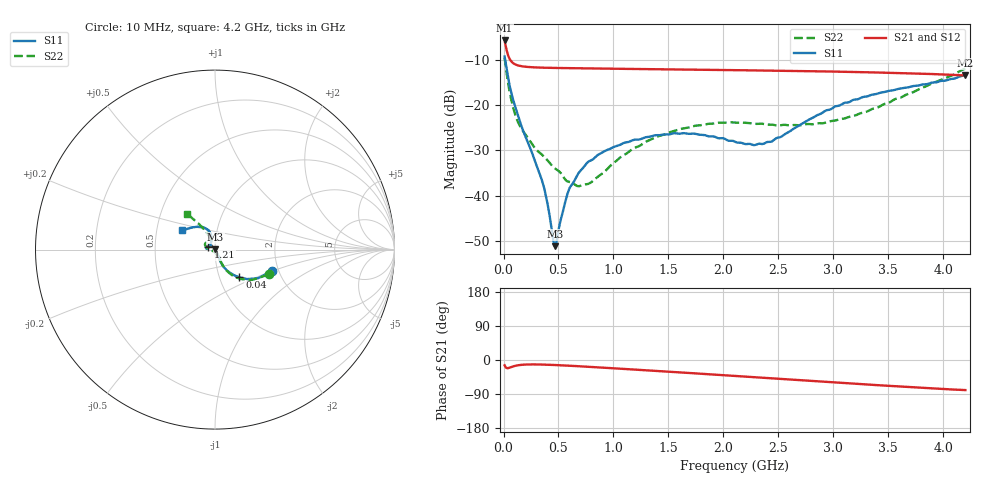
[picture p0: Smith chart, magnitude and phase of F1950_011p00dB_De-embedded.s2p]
! Integrated Device Technology
! Corporate Headquarters
! 6024 Silver Creek Valley Road
! San Jose, CA 95138  USA
! Phone:  1-408-284-8200
! Toll Free:  1-800-223-1366
! Webpage:  http://www.idt.com/
! Timing and RF Division
! 515 Groton Road, Suite 102
! Westford, MA 01886-6024
! Device:  F1950
! Description: 7-bit 0.25 dB Digital Step Attenuator
! Frequency:  150.0 -  4000.00 MHz
! Package:  4x4 mm Thin QFN Plastic Package: 24 pin
! Ports:  2 RF, 12 DC
!  Pin  1  = D0
!  Pin  2  = VDD
!  Pin  3  = Vmode
!  Pin  4  = GND
!  Pin  5  = RF1  =  Port 1
!  Pin  6  = GND
!  Pin  7  = GND
!  Pin  8  = GND
!  Pin  9  = GND
!  Pin 10  = GND
!  Pin 11  = GND
!  Pin 12  = GND
!  Pin 13  = GND
!  Pin 14  = RF2  =  Port 2
!  Pin 15  = GND
!  Pin 16  = LE
!  Pin 17  = CLK
!  Pin 18  = DATE
!  Pin 19  = D6
!  Pin 20  = D5
!  Pin 21  = D4
!  Pin 22  = D3
!  Pin 23  = D2
!  Pin 24  = D1
! State:  44
! Atten State:  11.00 dB
! Voltage:  +5.00 Volts
! Current:  Not Measured mA
! Data:  The device was measured on a the F195X evaluation board which has
!  individual transmission lines to the RF pins.  Data was collected
!  using a calibrated network analyzer.  The evaluation board was
!  de-embedded using a TRL calibration technique.
!  The reference plane is the edge of the package pin.
! Misc:  Board 2019
!  Action Tracker AT0250
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# GHz S dB R 50
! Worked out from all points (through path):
!   420 points, 10 MHz to 4.2 GHz, reference 50 ohm
!   highest |S21| = -5.80 dB at 10 MHz (marker M1); lowest = -13.5 dB at 4.2 GHz (marker M2)
!   group delay of S21, straight-line fit = 48.5 ps
!   lowest |S11| = -51.0 dB at 470 MHz (marker M3), VSWR 1.01, Z = 50.2 + j0.171 ohm
!   |S11| at or under -10 dB: 14.51 MHz to end of sweep
!   |S22| runs from -37.8 to -9.6 dB; largest |S21 - S12| = 0.00034
!   S11 on the Smith chart (normalised r, x): 10 MHz: 1.86, -0.49; 40 MHz: 1.24, -0.40; 1.21 GHz: 0.93, +0.03; 4.2 GHz: 0.68, +0.15
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0.01  -9.35 -20.2  -5.80 -14.0  -5.80 -14.0  -9.62 -24.8
0.04  -13.73 -48.7  -8.94 -21.5  -8.94 -21.5  -14.89 -55.2
0.09  -19.07 -63.1  -10.83 -16.7  -10.83 -16.7  -20.78 -63.5
0.15  -23.72 -65.5  -11.40 -13.2  -11.40 -13.2  -24.65 -65.6
0.35  -36.62 -51.0  -11.78 -12.0  -11.78 -12.0  -30.91 -71.1
0.4  -41.66 -41.3  -11.81 -12.5  -11.81 -12.5  -32.16 -71.6
0.45  -49.42 -5.4  -11.84 -13.0  -11.84 -13.0  -33.59 -76.5
0.47  -51.04 37.4  -11.85 -13.3  -11.85 -13.3  -34.00 -79.8
0.49  -48.88 75.8  -11.86 -13.5  -11.85 -13.5  -34.31 -82.1
0.59  -38.93 118.4  -11.89 -15.0  -11.89 -15.0  -36.84 -97.4
0.71  -34.20 129.5  -11.93 -16.9  -11.93 -16.9  -37.66 -124.2
0.91  -30.30 141.6  -11.99 -20.3  -11.99 -20.3  -34.86 -165.6
1.21  -27.61 157.3  -12.08 -25.6  -12.07 -25.6  -29.26 173.1
1.41  -26.63 165.7  -12.13 -29.2  -12.13 -29.2  -26.85 166.0
1.73  -26.29 173.3  -12.22 -35.0  -12.22 -35.0  -24.63 157.8
2.11  -28.13 164.3  -12.33 -42.2  -12.33 -42.2  -23.89 148.0
2.28  -28.83 146.7  -12.38 -45.3  -12.38 -45.4  -24.11 142.4
2.43  -28.09 128.8  -12.44 -48.1  -12.43 -48.1  -24.30 137.1
2.81  -22.84 105.4  -12.57 -55.3  -12.57 -55.4  -24.23 121.0
3.1  -19.52 107.6  -12.69 -60.8  -12.69 -60.9  -22.96 115.2
3.51  -16.86 119.2  -12.91 -68.3  -12.91 -68.4  -19.42 116.0
4.2  -13.41 149.3  -13.50 -79.4  -13.50 -79.4  -11.98 127.9
